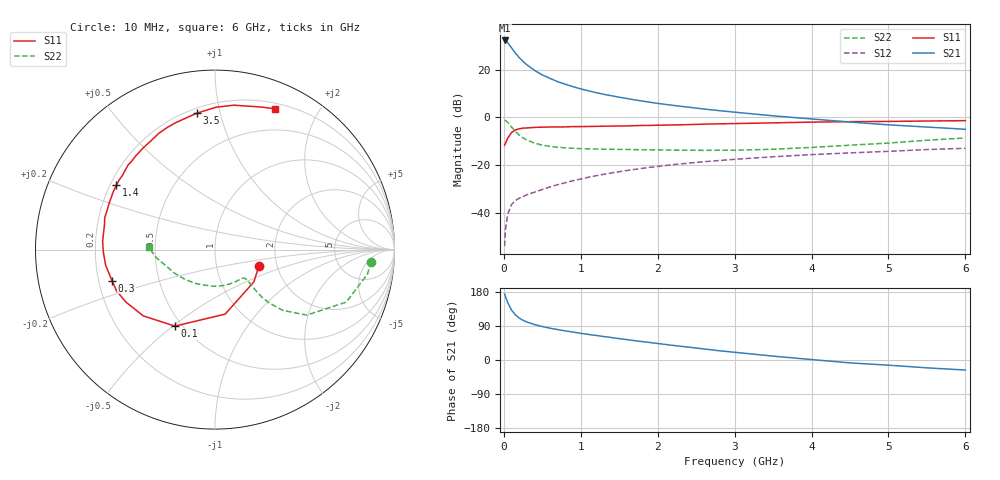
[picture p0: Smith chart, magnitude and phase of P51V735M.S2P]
! SIEMENS Small Signal Semiconductors
! BFP183
! Si NPN RF Bipolar Junction Transistor in SOT143
! VCE = 1.75 V  IC = 35 mA
! Common Emitter S-Parameters:  March  1996
# GHz  S  MA  R  50
!  f  S11  S21  S12  S22
! GHz  MAG  ANG  MAG  ANG  MAG  ANG  MAG  ANG
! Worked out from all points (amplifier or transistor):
!   36 points, 10 MHz to 6 GHz, reference 50 ohm
!   highest |S21| = 32.2 dB at 10 MHz (marker M1)
!   |S21| within 3 dB of that: start of sweep to 97.25 MHz
!   unconditionally stable (mu >= 1): start of sweep to 13.71 MHz; 369.4 MHz to end of sweep
!   at 250 MHz: K = 0.80, MSG = 28.3 dB, |S12| = -33.2 dB
!   at 1.4 GHz: K = 1.37, MAG = 12.5 dB, |S12| = -23.3 dB
!   at 6 GHz: K = 1.08, MAG = 2.3 dB, |S12| = -13.0 dB
!   S11 on the Smith chart (normalised r, x): 10 MHz: 1.61, -0.31; 100 MHz: 0.46, -0.51; 300 MHz: 0.26, -0.14; 1.4 GHz: 0.23, +0.28; 3.5 GHz: 0.23, +0.85; 6 GHz: 0.26, +1.48
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0.01  0.2613 -20.2  40.79 174.0  0.002 75.8  0.8726 -4.4
0.02  0.2815 -39.7  40.39 168.2  0.0043 76.1  0.8603 -9.2
0.05  0.3637 -81.0  36.8 151.4  0.0094 69.8  0.7876 -21.8
0.1  0.481 -117.6  28.47 131.7  0.0149 54.5  0.6282 -35.5
0.15  0.5441 -137.2  22.22 119.1  0.0181 48.9  0.507 -41.9
0.2  0.5753 -149.3  17.84 110.7  0.0202 47.7  0.4246 -44.5
0.25  0.5946 -157.0  14.78 104.7  0.0219 49.0  0.3706 -45.4
0.3  0.5995 -163.3  12.58 100.4  0.024 49.5  0.3332 -45.2
0.4  0.6157 -172.0  9.616 93.4  0.0271 51.5  0.2878 -44.5
0.5  0.6224 -178.8  7.73 88.3  0.0308 53.3  0.2613 -43.8
0.6  0.6276 176.0  6.551 84.0  0.0348 55.6  0.2461 -43.5
0.7  0.6279 171.3  5.586 80.2  0.0389 56.9  0.2361 -43.6
0.8  0.6311 167.2  4.93 76.8  0.0426 57.5  0.2299 -44.2
1.1  0.6442 156.2  3.592 67.4  0.0556 58.7  0.2183 -47.9
1.4  0.6559 146.9  2.833 59.3  0.0686 57.9  0.2138 -53.4
1.7  0.6686 138.2  2.318 51.0  0.0812 55.8  0.2109 -60.2
2.2  0.6935 125.3  1.782 38.5  0.102 51.8  0.2058 -73.5
2.8  0.7308 111.2  1.381 24.4  0.1245 45.9  0.2045 -92.7
3.5  0.7667 97.6  1.076 10.2  0.1492 39.3  0.2148 -116.9
4.5  0.8114 82.6  0.797 -7.6  0.1799 29.5  0.2607 -149.6
5.5  0.8369 71.5  0.626 -20.7  0.2116 20.7  0.331 -172.4
6  0.8522 66.9  0.562 -26.5  0.2245 15.7  0.3702 177.8
